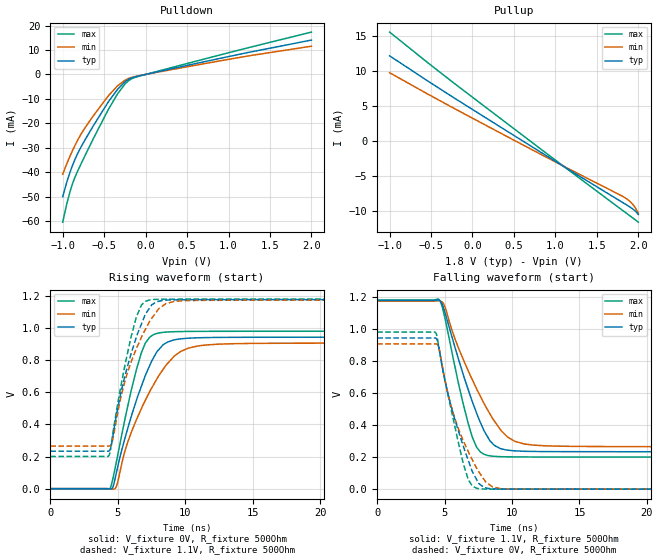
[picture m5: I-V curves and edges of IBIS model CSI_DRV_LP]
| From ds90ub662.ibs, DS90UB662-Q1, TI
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|   CSI_DRV_HS  Model
[Model]   CSI_DRV_LP
Model_type   Output
Polarity   Non-Inverting
Vmeas = 0.5
Vref = 0
Cref = 1pF
Rref = 100000
|   typ   min   max
C_comp   0.533pF   0.500pF   0.567pF
[Voltage Range]   1.8   1.71   1.89
[Temperature Range]   27   105   -40
[Pullup Reference]   1.8   1.71   1.89
[Pulldown Reference]   0   0   0
[Power Clamp Reference]   1.8   1.71   1.89
[GND Clamp Reference]   0   0   0
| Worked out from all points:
|   slope of the pulldown table from 0 to 0.27 V, typ, clamps not added: 135 ohm
|   slope of the pullup table from 0 to 0.27 V, typ, clamps not added: 134 ohm
|   falling waveform, V_fixture 1.1V, R_fixture 500Ohm: 20-80 % time 2.21ns typ, 2.97ns min, 1.57ns max; typ from 1.18 V to 0.234 V
|   rising waveform, V_fixture 0V, R_fixture 500Ohm: 20-80 % time 2.16ns typ, 2.85ns min, 1.57ns max; typ from 0 V to 0.944 V
|   rising waveform, V_fixture 1.1V, R_fixture 500Ohm: 20-80 % time 1.76ns typ, 2.11ns min, 1.38ns max; typ from 0.234 V to 1.18 V
|   falling waveform, V_fixture 0V, R_fixture 500Ohm: 20-80 % time 1.87ns typ, 2.14ns min, 1.5ns max; typ from 0.944 V to 0 V
[Pulldown]
|   Voltage   I(typ)   I(min)   I(max)
-1V       -50.05mA   -40.89mA   -60.49mA
-955mV    -44.55mA   -36.92mA   -53.6mA
-910mV    -39.84mA   -33.29mA   -47.77mA
-874mV    -36.58mA   -30.6mA    -44.02mA
-820mV    -32.38mA   -26.91mA   -39.59mA
-628mV    -20.87mA   -16.79mA   -26.1mA
-436mV    -10.58mA   -8.234mA   -13.55mA
-337mV    -6.05mA    -4.634mA   -7.893mA
-205mV    -2.028mA   -1.664mA   -2.569mA
-37mV     -278.5uA   -239.9uA   -334uA
1.22V     8.863mA    7.459mA    10.78mA
2V        14.07mA    11.55mA    17.33mA
[Pullup]
|   Voltage   I(typ)   I(min)   I(max)
-1V       12.13mA    9.717mA    15.52mA
-250mV    6.325mA    4.795mA    8.469mA
860mV     -1.919mA   -2.171mA   -1.524mA
1.814V    -8.859mA   -7.982mA   -10mA
1.916V    -9.62mA    -8.874mA   -10.9mA
1.958V    -10.01mA   -9.499mA   -11.27mA
2V        -10.55mA   -10.37mA   -11.65mA
[Ramp]
R_load = 500
|   typ   min   max
dV/dt_r   0.566411/2.16257e-09   0.544254/2.84929e-09   0.588619/1.56516e-09
dV/dt_f   0.566858/2.20908e-09   0.545657/2.97308e-09   0.588581/1.56746e-09
[Falling Waveform]
V_fixture = 1.1V
V_fixture_min = 1.1V
V_fixture_max = 1.1V
R_fixture = 500Ohm
C_fixture = 0F
|   Time   V(typ)   V(min)   V(max)
0s        1.178V     1.175V     1.182V
4.604ns   1.179V     1.177V     1.183V
4.995ns   1.112V     1.146V     1.079V
6.373ns   718.3mV    812.5mV    534.9mV
7.052ns   546.6mV    684.2mV    325.1mV
7.669ns   413.8mV    577.3mV    231.3mV
8.212ns   323.3mV    491.6mV    210.2mV
9.658ns   243.9mV    326.2mV    202mV
11.6ns    235.6mV    275mV      201mV
40ns      233.6mV    265.3mV    200.6mV
[Rising Waveform]
V_fixture = 0V
V_fixture_min = 0V
V_fixture_max = 0V
R_fixture = 500Ohm
C_fixture = 0F
|   Time   V(typ)   V(min)   V(max)
0s        89.58uV    227.2uV    28.13uV
4.439ns   -1.336mV   -929.4uV   3.109mV
4.896ns   97.15mV    13.05mV    165mV
5.599ns   333.2mV    252.5mV    458.9mV
6.758ns   638.8mV    499.4mV    847.9mV
7.38ns    769mV      606.6mV    944.8mV
7.932ns   856mV      687.9mV    968.1mV
9.658ns   933.5mV    854.7mV    979.2mV
11.6ns    941.6mV    895.8mV    980.5mV
40ns      944.1mV    907.3mV    981.1mV
[Rising Waveform]
V_fixture = 1.1V
V_fixture_min = 1.1V
V_fixture_max = 1.1V
R_fixture = 500Ohm
C_fixture = 0F
|   Time   V(typ)   V(min)   V(max)
0s        233.6mV    265.3mV    200.6mV
4.34ns    234.6mV    265.4mV    205.2mV
4.62ns    316.1mV    301.6mV    334mV
5.351ns   639.6mV    610.7mV    691.2mV
6.373ns   941.6mV    871.1mV    1.068V
6.758ns   1.026V     943.1mV    1.144V
7.38ns    1.128V     1.044V     1.176V
8.56ns    1.175V     1.153V     1.181V
9.658ns   1.177V     1.17V      1.181V
40ns      1.178V     1.175V     1.182V
[Falling Waveform]
|Gnd
V_fixture = 0V
V_fixture_min = 0V
V_fixture_max = 0V
R_fixture = 500Ohm
C_fixture = 0F
|   Time   V(typ)   V(min)   V(max)
0s        944.1mV    907.3mV    981.1mV
4.34ns    943.3mV    907.6mV    976.9mV
4.62ns    861.8mV    867.8mV    864mV
5.314ns   572.7mV    574.9mV    565.7mV
6.373ns   272.4mV    305mV      163.7mV
6.758ns   179.7mV    234.1mV    58.95mV
7.38ns    58.78mV    129.6mV    5.397mV
8.052ns   8.515mV    44.51mV    824.1uV
9.181ns   737.5uV    3.032mV    222.3uV
40ns      89.66uV    227.7uV    28.3uV
